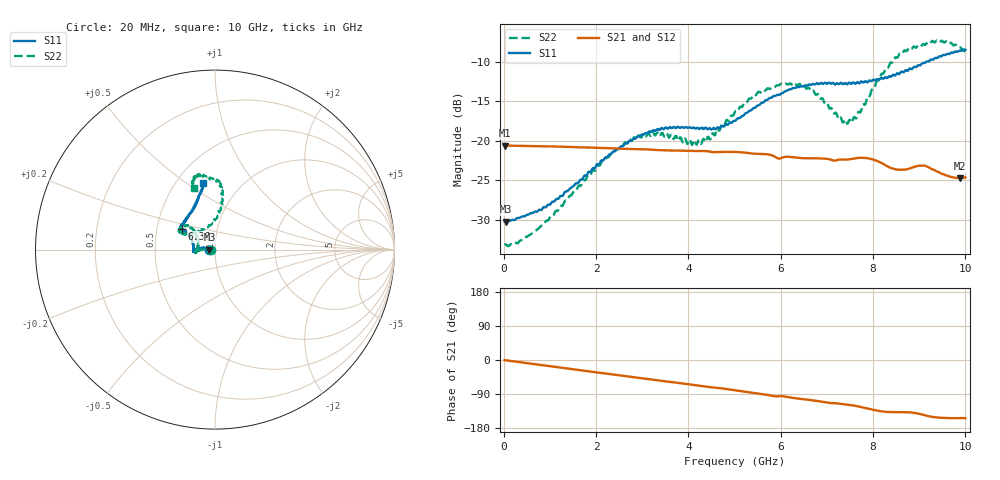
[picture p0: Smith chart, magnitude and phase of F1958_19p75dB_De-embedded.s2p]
! Integrated Device Technology
! Corporate Headquarters
! 6024 Silver Creek Valley Road
! San Jose, CA 95138  USA
! Phone:  1-408-284-8200
! Toll Free:  1-800-223-1366
! Webpage:  http://www.idt.com/
! Timing and RF Division
! 515 Groton Road, Suite 102
! Westford, MA 01886-6024
! Device:  F1958
! Description: 7-bit 0.25 dB Digital Step Attenuator
! Frequency:  0.001 -  6.000 GHz
! Package:  4x4 mm Thin QFN Plastic Package: 24 pin
! Ports:  2 RF, 12 DC
!  Pin  1  = D0
!  Pin  2  = VDD
!  Pin  3  = VMODE
!  Pin  4  = GND
!  Pin  5  = RF1  =  Port 1
!  Pin  6  = GND
!  Pin  7  = GND
!  Pin  8  = GND
!  Pin  9  = GND
!  Pin 10  = GND
!  Pin 11  = GND
!  Pin 12  = GND
!  Pin 13  = GND
!  Pin 14  = RF2  =  Port 2
!  Pin 15  = GND
!  Pin 16  = LE
!  Pin 17  = CLK
!  Pin 18  = DATA
!  Pin 19  = D6
!  Pin 20  = D5
!  Pin 21  = D4
!  Pin 22  = D3
!  Pin 23  = D2
!  Pin 24  = D1
! State:  79
! Atten State:  19.75 dB
! Voltage:  +3.30 Volts
! Current:  0.257 mA
! Data:  The device was measured on a F1958 evaluation board which has
!  individual transmission lines to the RF pins.  Data was collected
!  using a calibrated network analyzer.  The evaluation board was
!  de-embedded using Automatic Fixture Removal (AFR).
!  The reference plane is the edge of the package pin.
! Misc:
!  Action Tracker AT0419
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# GHz S dB R 50
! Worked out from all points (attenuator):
!   500 points, 20 MHz to 10 GHz, reference 50 ohm
!   highest |S21| = -20.63 dB at 20 MHz (marker M1); lowest = -24.8 dB at 9.88 GHz (marker M2)
!   lowest |S11| = -30.3 dB at 40 MHz (marker M3), VSWR 1.06, Z = 47 - j0.0445 ohm
!   |S11| at or under -10 dB: start of sweep to 9.155 GHz
!   |S22| runs from -33.4 to -7.3 dB; largest |S21 - S12| = 0.00042
!   S11 on the Smith chart (normalised r, x): 20 MHz: 0.94, -0.00; 6.36 GHz: 0.67, +0.16; 10 GHz: 0.68, +0.58
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0.02  -30.23 -178.9  -20.63 -0.4  -20.63 -0.4  -33.21 -178.0
0.04  -30.26 -179.1  -20.64 -0.7  -20.63 -0.7  -33.13 -177.0
0.32  -29.79 175.1  -20.67 -5.4  -20.66 -5.4  -32.90 179.2
0.72  -29.01 172.6  -20.71 -11.9  -20.70 -11.8  -31.29 -179.7
1.7  -24.90 171.1  -20.86 -27.6  -20.86 -27.6  -25.32 179.2
2.6  -20.61 177.0  -21.04 -41.9  -21.02 -41.9  -20.46 -177.0
3.36  -18.63 -175.5  -21.21 -54.1  -21.21 -54.2  -19.27 -169.9
4.24  -18.54 -178.9  -21.32 -67.6  -21.33 -67.7  -20.00 167.8
4.5  -18.61 175.2  -21.44 -72.2  -21.45 -72.2  -19.41 152.1
5.02  -17.48 160.8  -21.44 -80.0  -21.45 -80.0  -16.27 138.6
5.58  -15.23 150.6  -21.70 -89.5  -21.71 -89.5  -13.82 138.8
6.36  -13.21 148.1  -22.17 -101.6  -22.19 -101.5  -13.05 151.9
6.68  -12.87 146.6  -22.24 -106.2  -22.26 -106.1  -13.72 152.8
7.3  -12.68 141.0  -22.40 -115.7  -22.41 -115.6  -17.05 131.6
7.5  -12.71 138.4  -22.36 -118.8  -22.36 -118.7  -17.37 113.3
7.68  -12.67 135.5  -22.19 -122.5  -22.19 -122.5  -16.38 96.4
7.92  -12.37 129.3  -22.29 -129.1  -22.28 -129.1  -14.39 86.3
8.34  -11.88 119.4  -23.34 -137.4  -23.34 -137.5  -10.64 81.6
8.68  -11.24 112.7  -23.67 -137.6  -23.69 -137.5  -8.57 86.1
9.26  -9.73 105.0  -23.58 -149.8  -23.56 -149.9  -7.51 99.0
9.88  -8.61 100.4  -24.75 -153.3  -24.78 -153.4  -8.20 108.2
10  -8.51 100.0  -24.66 -153.7  -24.71 -153.6  -8.75 108.8
